(* Logix 5000 AddOnInstructionDefinition export AMP_Input_Assembly; software revision 20.04 *)

TYPE AMP_Status_Word :   // Applied Motion Input Assembly Status Word
STRUCT
   Enabled : BOOL;   // Motor Enabled (Motor Disabled if this bit = 0)
   Sampling : BOOL;   // Sampling (for Quick Tuner)
   Drive_Fault : BOOL;   // Drive Fault (check Alarm Code)
   In_Position : BOOL;   // In Position (motor is in position)
   Moving : BOOL;   // Moving (motor is moving)
   Jogging : BOOL;   // Jogging (currently in jog mode)
   Stopping : BOOL;   // Stopping (in the process of stopping from a stop command)
   Waiting : BOOL;   // Waiting (for an input; executing a WI command)
   Saving : BOOL;   // Saving (parameter data is being saved)
   Alarm_Present : BOOL;   // Alarm present (check Alarm Code)
   Homing : BOOL;   // Homing (executing an SH command)
   Wait_Time : BOOL;   // Waiting (for time; executing a WD or WT command)
   Wizard_Running : BOOL;   // Wizard running (Timing Wizard is running)
   Checking_Encoder : BOOL;   // Checking encoder (Timing Wizard is running)
   Q_Program_Running : BOOL;   // Q Program is running
   Initializing : BOOL;   // Initializing (happens at power up) ; Servo Ready (for SV200 drives only)
END_STRUCT
END_TYPE

TYPE AMP_Input_Assembly_v2 :   // Applied Motion Drive Input Assembly Version 2.0
STRUCT
   Status_Code : DINT;   // Status Code
   Alarm_Code : DINT;   // Alarm Code
   Voltage : DINT;   // Supply Voltage (x0.1V)
   Current : DINT;   // Actual Current (mA)
   Temp : DINT;   // Drive Temperature (0.1 deg C)
   Encoder_Position : DINT;   // Encoder Position (20,000 counts = 1 shaft turn)
   Absolute_Position : DINT;   // Absolute Position (20,000 counts = 1 shaft turn)
   Position_Error : DINT;   // Position Error (counts)
   Actual_Velocity : DINT;   // Actual Velocity (rev/sec * 240, 0 when no encoder)
   Extended_Inputs : DINT;   // Input Status (Extended)
   Main_Board_Inputs : DINT;   // Input Status (Main board)
   Word11 : DINT;   // Reserved
   Analog_Input_1 : DINT;   // Analog Input 1 (ADC counts, 0=min V, 16383 = max V)
   Analog_Input_2 : DINT;   // Analog Input 2 (ADC counts, 0=min V, 16383 = max V)
END_STRUCT
END_TYPE

ADD_ON_INSTRUCTION AMP_Input_Assembly   (* revision 1.0 *)
// Applied Motion - Input Assembly AOI
// Help:
// The Input Assembly AOI takes raw input data from the drive and re-interprets the data, using either scaling or copying, to appropriately named outputs.
VAR_IN_OUT
   Input : DINT[14]; {required}   // AMP_Assembly
   Output : AMP_Input_Assembly_v2; {required}
END_VAR
VAR_OUTPUT
   Status_Code : DINT; {access Read Only, visible}   // Status Code
   Alarm_Code : DINT; {access Read Only, visible}   // Alarm Code
   Voltage : REAL; {access Read Only, visible}   // Supply Voltage (V)
   Current : REAL; {access Read Only, visible}   // Actual Current (mA)
   Temp : REAL; {access Read Only, visible}   // Drive Temperature (deg C)
   Encoder_Position : DINT; {access Read Only, visible}   // Encoder Position (20,000 counts = 1 shaft turn)
   Absolute_Position : DINT; {access Read Only, visible}   // Absolute Position (20,000 counts = 1 shaft turn)
   Actual_Velocity : REAL; {access Read Only, visible}   // Actual Velocity (rev/sec, 0 when no encoder)
   Position_Error : DINT; {access Read Only, visible}
   Extended_Inputs : INT; {access Read Only, visible}   // Input Status (Extended)
   Main_Board_Inputs : INT; {access Read Only, visible}   // Input Status (Main board)
   Analog_Input_1 : DINT; {access Read Only, visible}   // Analog Input 1 (ADC counts, 0=min V, 16383 = max V)
   Analog_Input_2 : DINT; {access Read Only, visible}   // Analog Input 2 (ADC counts, 0=min V, 16383 = max V)
END_VAR
VAR
   Loc_Input_Assembly : AMP_Input_Assembly_v2; {access None}
   Loc_StatusCode : AMP_Status_Word; {access None}
END_VAR

ROUTINE Logic   (* ladder *)
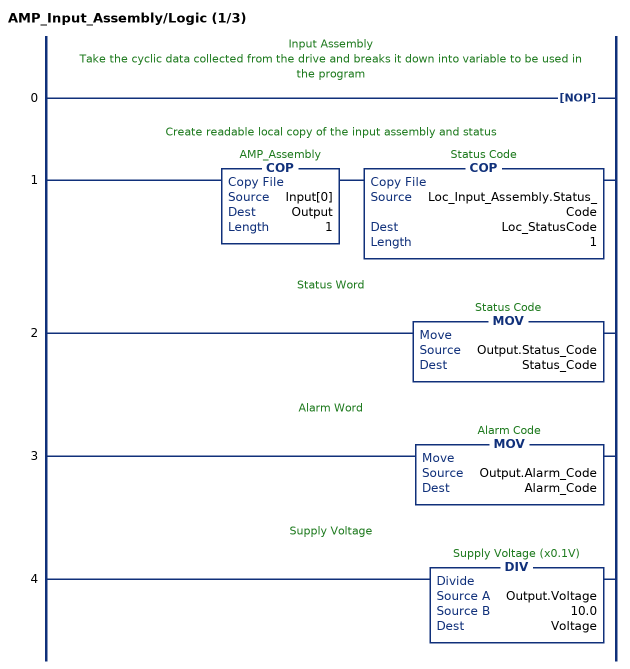
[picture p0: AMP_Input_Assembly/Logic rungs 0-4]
   // Input Assembly
   // Take the cyclic data collected from the drive and breaks it down into variable to be used in the program
   0: NOP();
   // Create readable local copy of the input assembly and status
   1: COP(Input[0],Output,1)COP(Loc_Input_Assembly.Status_Code,Loc_StatusCode,1);
   // Status Word
   2: MOV(Output.Status_Code,Status_Code);
   // Alarm Word
   3: MOV(Output.Alarm_Code,Alarm_Code);
   // Supply Voltage
   4: DIV(Output.Voltage,10.0,Voltage);
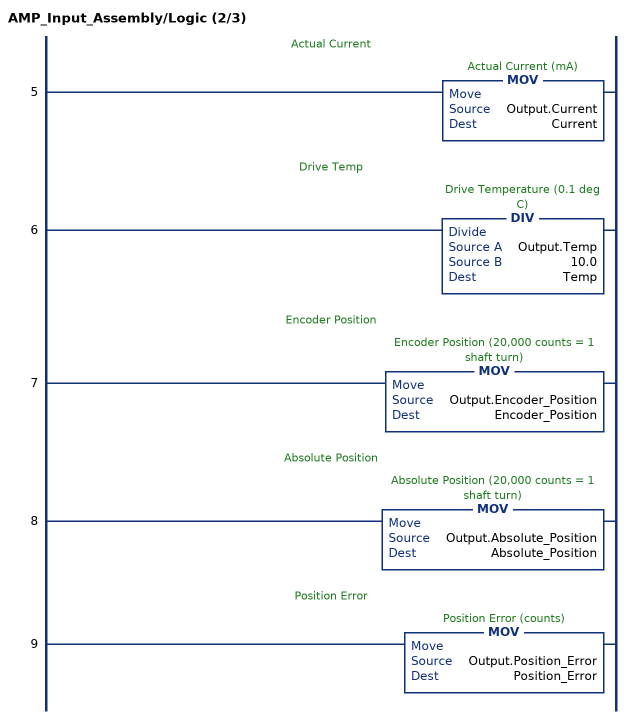
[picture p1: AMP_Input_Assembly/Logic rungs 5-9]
   // Actual Current
   5: MOV(Output.Current,Current);
   // Drive Temp
   6: DIV(Output.Temp,10.0,Temp);
   // Encoder Position
   7: MOV(Output.Encoder_Position,Encoder_Position);
   // Absolute Position
   8: MOV(Output.Absolute_Position,Absolute_Position);
   // Position Error
   9: MOV(Output.Position_Error,Position_Error);
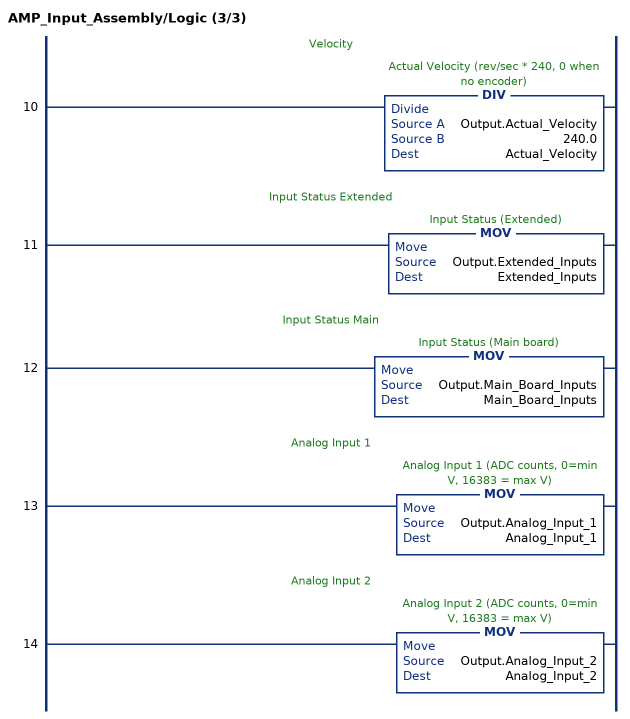
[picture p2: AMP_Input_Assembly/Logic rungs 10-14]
   // Velocity
   10: DIV(Output.Actual_Velocity,240.0,Actual_Velocity);
   // Input Status Extended
   11: MOV(Output.Extended_Inputs,Extended_Inputs);
   // Input Status Main
   12: MOV(Output.Main_Board_Inputs,Main_Board_Inputs);
   // Analog Input 1
   13: MOV(Output.Analog_Input_1,Analog_Input_1);
   // Analog Input 2
   14: MOV(Output.Analog_Input_2,Analog_Input_2);
END_ROUTINE
END_ADD_ON_INSTRUCTION
